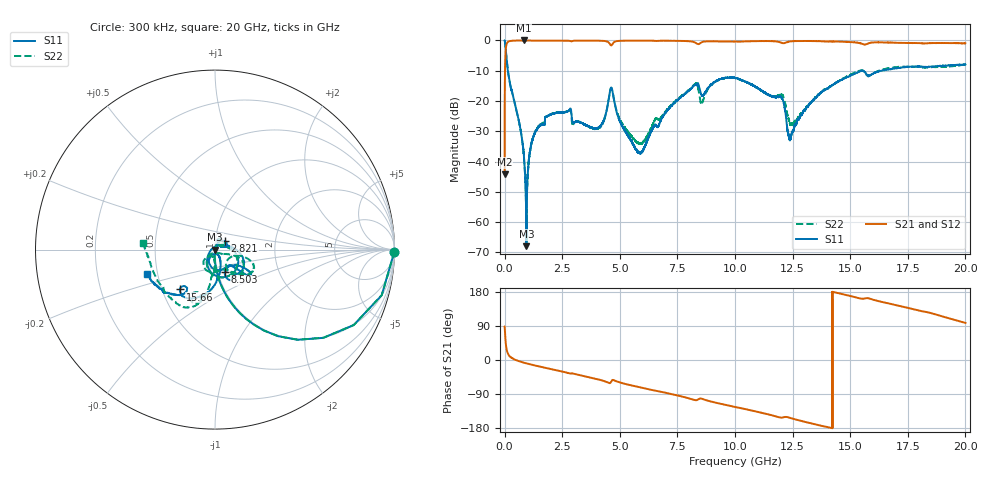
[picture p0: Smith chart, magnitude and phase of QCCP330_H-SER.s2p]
!{QCCP330}
!Johanson Technology Inc.
!www.johansontechnology.com
!Test Board Conditions:
!Substrate Type  RO4350B
!Substrate Thickness  20 mil
!Substrate Dk  3.66
!TL Type: GCPW
!TL Trace Width  36 mil
!TL Gap  12 mil
!Electrode orientation  Horizontal
!DUT TOPOLOGY	SERIES
!Mounting Pad LxW  26x36 mil
! Created Sat Jan  9 18:35:36 2021
# hz S ma R 50
! 2 Port Network Data from SP1.SP block
! freq  magS11  angS11  magS21  angS21  magS12  angS12  magS22  angS22
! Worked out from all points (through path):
!   20001 points, 300 kHz to 20 GHz, reference 50 ohm
!   highest |S21| = -0.01 dB at 820.3 MHz (marker M1); lowest = -44.2 dB at 300 kHz (marker M2)
!   group delay of S21, straight-line fit = 36.2 ps
!   lowest |S11| = -68.0 dB at 947.3 MHz (marker M3), VSWR 1.00, Z = 50 + j0.01 ohm
!   |S11| at or under -10 dB: 143.3 MHz to 15.53 GHz (15.39 GHz wide, 196 % of centre); 15.53628 GHz to 15.53818 GHz (1.901 MHz wide, 0.0122 % of centre); 15.56 GHz to 16.37 GHz (808.3 MHz wide, 5.06 % of centre)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
!   |S22| runs from -61.4 to 0.0 dB; largest |S21 - S12| = 0.017
!   S11 on the Smith chart (normalised r, x): 300 kHz: open; 2.821 GHz: 1.11, +0.11; 8.503 GHz: 1.08, -0.28; 15.66 GHz: 0.62, -0.30; 20 GHz: 0.44, -0.14
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300000  0.9989 -0.7  0.006197 88.2  0.006174 89.6  1 -0.7
1.273e8  0.3531 -70.3  0.9325 19.4  0.9337 19.4  0.3544 -70.3
8.203e8  0.01473 -94.3  0.999 -6.8  0.9984 -6.8  0.01512 -93.0
9.473e8  0.0004 14.5  0.9975 -8.9  0.9977 -8.8  0.001018 2.6
1.1503e9  0.01864 75.0  0.9978 -12.0  0.9975 -12.0  0.01885 75.0
1.3843e9  0.03342 71.6  0.9968 -15.4  0.9968 -15.3  0.03421 73.4
2.8213e9  0.07258 40.5  0.9852 -35.3  0.9847 -35.3  0.07082 55.4
3.3343e9  0.04359 37.4  0.9938 -41.0  0.9938 -41.0  0.04348 58.6
4.1473e9  0.03818 26.4  0.9889 -52.5  0.9886 -52.5  0.03694 34.5
4.6303e9  0.166 -59.2  0.8277 -56.4  0.8275 -56.4  0.1657 -62.1
5.0653e9  0.04117 -146.3  0.9881 -60.4  0.9868 -60.5  0.04439 -136.0
5.8193e9  0.01407 135.4  0.9935 -71.3  0.9936 -71.3  0.01977 -97.0
6.6673e9  0.03795 27.1  0.9846 -82.2  0.9829 -82.1  0.04975 -37.8
8.2653e9  0.1844 -30.8  0.9232 -105.7  0.9225 -105.7  0.1911 -33.9
8.5033e9  0.1375 -66.8  0.909 -101.6  0.9069 -101.5  0.09702 -51.0
1.00003e10  0.2407 -36.7  0.9603 -124.0  0.9589 -124.0  0.2397 -32.5
1.20043e10  0.1155 -81.1  0.9211 -152.0  0.9219 -152.0  0.1283 -100.0
1.23803e10  0.02267 -83.3  0.9627 -152.6  0.9636 -152.4  0.04237 -124.7
1.33343e10  0.09861 -71.9  0.9773 -167.6  0.9796 -167.6  0.09887 -91.9
1.56553e10  0.2953 -131.3  0.8582 162.7  0.865 162.3  0.2852 -118.0
1.66673e10  0.3318 -131.2  0.9239 149.2  0.9135 149.0  0.3485 -112.6
2e10  0.4003 -160.6  0.8957 97.8  0.8847 97.7  0.4035 174.9
